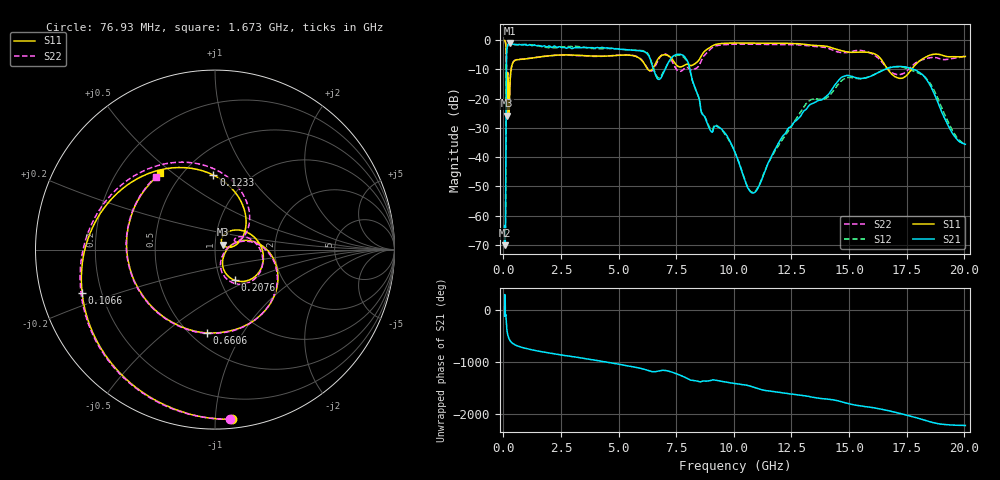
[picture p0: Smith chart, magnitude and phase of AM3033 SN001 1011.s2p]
# Hz S DB R 50
!freq MagS11 AngS11 MagS21 AngS21 MagS12 AngS12 MagS22 AngS22
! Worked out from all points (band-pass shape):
!   1601 points, 50 MHz to 20.05 GHz, reference 50 ohm
!   highest |S21| = -0.99 dB at 263.8 MHz (marker M1); lowest = -70.2 dB at 50 MHz (marker M2)
!   |S21| within 3 dB of the highest: 138.1 MHz to 6.127 GHz (5.988 GHz wide, 191 % of centre)
!   lowest |S11| = -25.8 dB at 140.1 MHz (marker M3), VSWR 1.11, Z = 54.4 + j3.04 ohm
!   |S11| at or under -10 dB: 126.4 MHz to 333.2 MHz (206.8 MHz wide, 90 % of centre); 6.264 GHz to 6.457 GHz (193 MHz wide, 3.03 % of centre); 16.68 GHz to 17.71 GHz (1.027 GHz wide, 5.97 % of centre)
!   |S22| runs from -25.5 to -0.1 dB; largest |S21 - S12| = 0.064
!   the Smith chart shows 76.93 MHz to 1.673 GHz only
!   S11 on the Smith chart (normalised r, x): 76.93 MHz: 0.06, -1.10; 106.6 MHz: 0.13, -0.16; 123.3 MHz: 0.70, +0.70; 207.6 MHz: 1.17, -0.42; 660.6 MHz: 0.60, -0.71; 1.673 GHz: 0.39, +0.45
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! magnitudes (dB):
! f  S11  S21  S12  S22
! 50 MHz  -0.1  -70.2  -65.5  -0.1
! 76.93 MHz  -0.4  -68.2  -69.7  -0.5
! 90.37 MHz  -0.9  -62.4  -61.3  -0.9
! 106.6 MHz  -2.2  -34.2  -34.3  -2.2
! 123.3 MHz  -7.6  -11.1  -11.1  -7.1
! 135.9 MHz  -22.4  -4.4  -4.4  -16.8
! 140.1 MHz  -25.8  -3.7  -3.7  -18.4
! 165.2 MHz  -12.2  -2.3  -2.3  -11.8
! 207.6 MHz  -13.9  -1.4  -1.4  -14.0
! 242.1 MHz  -24.5  -1.0  -1.0  -25.4
! 263.8 MHz  -19.3  -1.0  -1.0  -19.3
! 369.6 MHz  -8.6  -1.3  -1.3  -8.5
! 660.6 MHz  -6.6  -1.5  -1.5  -6.6
! 1.005 GHz  -6.4  -1.8  -1.5  -6.4
! 1.673 GHz  -5.6  -2.2  -2.3  -5.6
! 2.722 GHz  -5.1  -2.8  -2.4  -5.1
! 7.402 GHz  -7.4  -5.3  -5.7  -8.6
! 10.81 GHz  -1.1  -52.3  -52.1  -1.4
! 13.18 GHz  -1.6  -23.3  -21.5  -1.9
! 16.88 GHz  -11.8  -9.2  -9.1  -11.2
! 18.12 GHz  -6.8  -11.4  -11.7  -6.9
! 20.05 GHz  -5.6  -35.6  -35.5  -5.3
